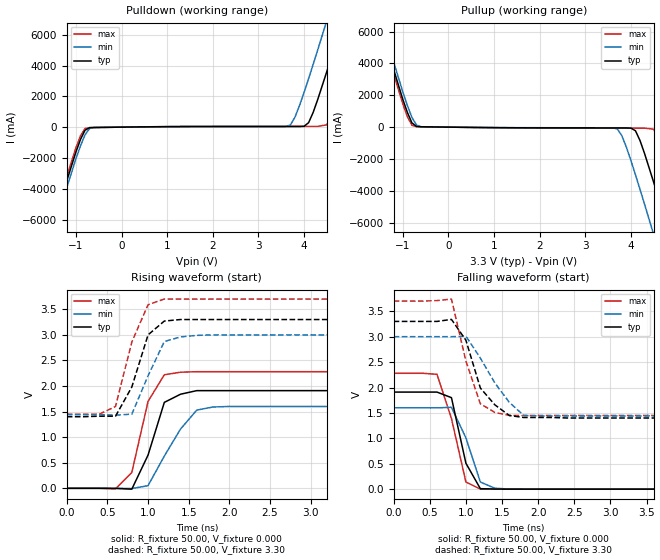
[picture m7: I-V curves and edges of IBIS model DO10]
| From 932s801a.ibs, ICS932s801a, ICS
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|   Model DO10
[Model]   DO10
Model_type   Output
Polarity   Non-Inverting
C_comp   5.50pF   5.00pF   6.00pF
[Temperature Range]   27.00   70.00   0.000
[Voltage Range]   3.30V   3.00V   3.70V
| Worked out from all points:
|   slope of the pulldown table from 0 to 0.495 V, typ, clamps not added: 27.2 ohm
|   slope of the pullup table from 0 to 0.495 V, typ, clamps not added: 29.2 ohm
|   rising waveform, R_fixture 50.00, V_fixture 0.000: 20-80 % time 251ps typ, 372ps min, 227ps max; typ from 0 V to 1.91 V
|   rising waveform, R_fixture 50.00, V_fixture 3.30: 20-80 % time 254ps typ, 265ps min, 259ps max; typ from 1.4 V to 3.3 V
|   falling waveform, R_fixture 50.00, V_fixture 0.000: 20-80 % time 209ps typ, 249ps min, 249ps max; typ from 1.91 V to 0 V
|   falling waveform, R_fixture 50.00, V_fixture 3.30: 20-80 % time 325ps typ, 428ps min, 267ps max; typ from 3.3 V to 1.4 V
[Pulldown]
| voltage   I(typ)   I(min)   I(max)
-3.3V     -24.04A    -24.44A    -23.66A
-1.7V     -8.19A     -8.63A     -7.92A
-1.5V     -6.26A     -6.71A     -5.99A
-800mV    -200mA     -500mA     -88.71mA
-600mV    -23.81mA   -23.75mA   -25.47mA
3.7V      41.14mA    140mA      50.72mA
4.1V      290mA      3.15A      50.89mA
4.5V      3.62A      6.93A      150mA
4.7V      5.51A      8.86A      1.51A
4.9V      7.44A      10.8A      3.33A
5.3V      11.33A     14.72A     7.15A
6.6V      24.16A     27.56A     19.93A
[Pullup]
| voltage   I(typ)   I(min)   I(max)
-3.3V     24.07A     24.51A     23.8A
-1.5V     6.42A      6.88A      6.12A
-1V       1.75A      2.22A      1.47A
-800mV    270mA      610mA      120mA
-600mV    23.66mA    25.86mA    25.64mA
3.7V      -50.36mA   -110mA     -63.36mA
4.1V      -230mA     -3A        -64.16mA
4.5V      -3.48A     -6.77A     -130mA
4.7V      -5.37A     -8.7A      -1.41A
4.9V      -7.3A      -10.64A    -3.21A
5.3V      -11.2A     -14.56A    -7.03A
6.6V      -24.04A    -27.41A    -19.83A
[Ramp]
| variable   typ   min   max
dV/dt_r   1.14/0.22n   0.96/0.26n   1.37/0.19n
dV/dt_f   1.14/0.27n   0.93/0.35n   1.35/0.23n
R_load = 50.00
[Rising Waveform]
R_fixture = 50.00
V_fixture = 0.000
V_fixture_min = 0.000
V_fixture_max = 0.000
| time   V(typ)   V(min)   V(max)
0s        0V         0V         0V
600ps     -1.64mV    640uV      -11.61mV
800ps     -16.54mV   -4.91mV    310mV
1ns       650mV      52.32mV    1.7V
1.2ns     1.68V      630mV      2.22V
1.4ns     1.84V      1.16V      2.27V
1.6ns     1.91V      1.53V      2.28V
1.8ns     1.91V      1.59V      2.28V
2ns       1.91V      1.6V       2.28V
10ns      1.91V      1.6V       2.28V
[Rising Waveform]
R_fixture = 50.00
V_fixture = 3.30
V_fixture_min = 3.00
V_fixture_max = 3.70
| time   V(typ)   V(min)   V(max)
0s        1.4V       1.44V      1.45V
400ps     1.41V      1.44V      1.45V
600ps     1.41V      1.43V      1.6V
800ps     1.98V      1.45V      2.86V
1ns       3V         2.2V       3.59V
1.2ns     3.27V      2.87V      3.7V
1.4ns     3.3V       2.96V      3.7V
1.6ns     3.3V       2.99V      3.7V
1.8ns     3.3V       3V         3.7V
10ns      3.3V       3V         3.7V
[Falling Waveform]
R_fixture = 50.00
V_fixture = 0.000
V_fixture_min = 0.000
V_fixture_max = 0.000
| time   V(typ)   V(min)   V(max)
0s        1.91V      1.6V       2.28V
400ps     1.91V      1.6V       2.28V
600ps     1.91V      1.6V       2.26V
800ps     1.8V       1.61V      1.39V
1ns       510mV      1.01V      140mV
1.2ns     9.62mV     140mV      1.73mV
1.4ns     2.49mV     17.75mV    740uV
1.6ns     520uV      2.27mV     120uV
10ns      -1.11uV    -740nV     0V
[Falling Waveform]
R_fixture = 50.00
V_fixture = 3.30
V_fixture_min = 3.00
V_fixture_max = 3.70
| time   V(typ)   V(min)   V(max)
0s        3.3V       3V         3.7V
600ps     3.3V       3V         3.71V
800ps     3.34V      3V         3.74V
1ns       2.93V      3.01V      2.52V
1.2ns     1.99V      2.58V      1.68V
1.4ns     1.66V      2.09V      1.51V
1.6ns     1.45V      1.71V      1.45V
1.8ns     1.41V      1.45V      1.45V
2ns       1.41V      1.44V      1.45V
10ns      1.4V       1.44V      1.45V
